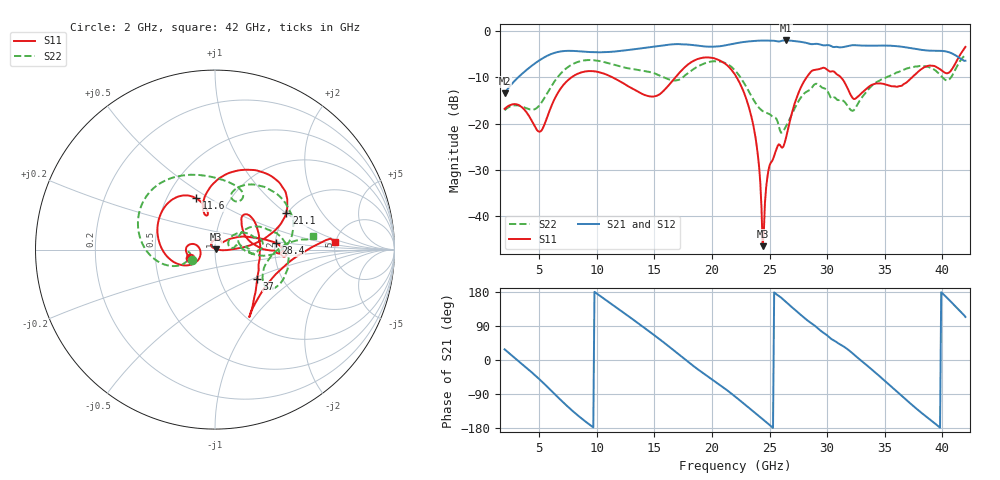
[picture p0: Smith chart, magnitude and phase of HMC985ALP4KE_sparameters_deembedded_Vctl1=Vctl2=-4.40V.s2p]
!s2p File: Measurements: S11, S21, S12, S22
# GHz S dB R 50.0
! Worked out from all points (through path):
!   401 points, 2 GHz to 42 GHz, reference 50 ohm
!   highest |S21| = -2.07 dB at 26.4 GHz (marker M1); lowest = -13.4 dB at 2 GHz (marker M2)
!   lowest |S11| = -46.4 dB at 24.4 GHz (marker M3), VSWR 1.01, Z = 50.4 + j0.255 ohm
!   |S11| at or under -10 dB: start of sweep to 7.823 GHz; 22.14 GHz to 28.22 GHz (6.086 GHz wide, 24.2 % of centre); 31.18 GHz to 37.38 GHz (6.2 GHz wide, 18.1 % of centre)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
!   |S22| runs from -22.0 to -5.2 dB; largest |S21 - S12| = 0.00068
!   S11 on the Smith chart (normalised r, x): 2 GHz: 0.76, -0.07; 11.6 GHz: 0.70, +0.44; 21.1 GHz: 1.98, +1.01; 28.4 GHz: 2.01, +0.17; 37 GHz: 1.50, -0.53; 42 GHz: 4.97, +0.72
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2  -16.82 -161.8  -13.44 28.2  -13.45 28.2  -17.12 -155.6
3.3  -16.11 173.3  -9.74 -5.3  -9.74 -5.3  -16.16 -173.4
5  -21.76 -173.4  -6.39 -50.2  -6.39 -50.2  -16.12 -160.3
6.3  -14.88 -150.7  -4.77 -88.5  -4.77 -88.5  -11.01 -162.0
8.7  -8.93 150.1  -4.44 -154.7  -4.45 -154.7  -6.46 151.0
11.6  -10.33 110.2  -4.45 140.7  -4.45 140.7  -7.38 103.2
13.6  -13.16 101.4  -3.85 96.8  -3.85 96.8  -8.43 75.4
15.4  -13.77 106.3  -3.25 56.0  -3.24 56.0  -9.56 62.0
17.9  -7.28 79.9  -2.95 -4.1  -2.95 -4.1  -9.15 72.0
21.1  -7.00 27.2  -3.15 -75.0  -3.15 -74.9  -6.89 15.6
22  -9.43 16.7  -2.71 -96.2  -2.71 -96.2  -8.52 0.2
23.6  -20.52 0.6  -2.18 -136.0  -2.18 -135.9  -14.85 -4.1
24.4  -46.45 32.0  -2.09 -156.1  -2.09 -156.1  -17.30 7.7
25  -29.02 129.6  -2.11 -171.4  -2.11 -171.4  -17.97 11.6
26.4  -23.35 41.6  -2.06 153.9  -2.06 153.9  -20.74 33.4
28.4  -9.38 6.4  -2.73 101.8  -2.73 101.8  -12.88 17.8
28.7  -8.58 1.4  -2.87 95.6  -2.87 95.6  -12.17 16.0
32.5  -14.53 33.3  -3.10 9.7  -3.10 9.7  -16.46 28.6
35.4  -11.78 18.4  -3.19 -65.8  -3.19 -65.7  -9.75 19.1
37  -10.88 -34.4  -3.61 -108.9  -3.61 -108.9  -8.06 4.4
39.8  -8.26 -56.8  -4.30 -178.7  -4.30 -178.7  -9.46 -35.3
42  -3.46 3.4  -6.45 113.6  -6.45 113.6  -5.22 8.0
